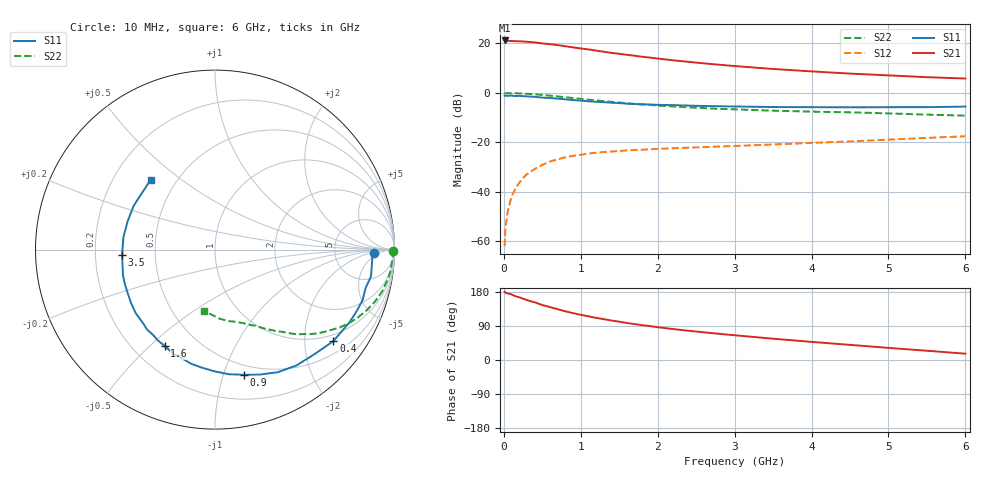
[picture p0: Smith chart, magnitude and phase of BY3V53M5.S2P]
! SIEMENS Small Signal Semiconductors
! BFY420
! Si NPN RF SIEGET Grounded Emitter Transistor in MICRO-X
! VCE = 3.5 V  IC = 3.5 mA
! Common Emitter S-Parameters:  October  1996
# GHz  S  MA  R  50
!  f  S11  S21  S12  S22
! GHz  MAG  ANG  MAG  ANG  MAG  ANG  MAG  ANG
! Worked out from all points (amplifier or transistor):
!   36 points, 10 MHz to 6 GHz, reference 50 ohm
!   highest |S21| = 21.2 dB at 10 MHz (marker M1)
!   |S21| within 3 dB of that: start of sweep to 945.6 MHz
!   unconditionally stable (mu >= 1): 3.471 GHz to end of sweep
!   at 250 MHz: K = 0.10, MSG = 27.6 dB, |S12| = -34.4 dB
!   at 1.4 GHz: K = 0.42, MSG = 19.9 dB, |S12| = -23.7 dB
!   at 6 GHz: K = 1.17, MAG = 9.2 dB, |S12| = -17.5 dB
!   S11 on the Smith chart (normalised r, x): 10 MHz: 16, -3; 400 MHz: 0.81, -2.71; 900 MHz: 0.41, -1.17; 1.6 GHz: 0.33, -0.56; 3.5 GHz: 0.32, -0.03; 6 GHz: 0.36, +0.39
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0.01  0.8833 -1.2  11.48 180.0  0.0008 66.2  0.9937 -0.5
0.02  0.878 -2.2  11.46 177.9  0.0018 66.5  0.9854 -0.8
0.05  0.8777 -4.7  11.24 175.6  0.004 79.9  0.9914 -2.3
0.1  0.8821 -9.7  11.2 173.0  0.008 83.2  0.9868 -4.7
0.15  0.8661 -14.3  11.12 168.3  0.0117 79.7  0.9847 -7.0
0.2  0.8691 -19.1  11.05 165.6  0.0152 77.5  0.9782 -9.3
0.3  0.8512 -28.5  10.8 158.2  0.0228 73.9  0.9613 -13.8
0.4  0.8336 -37.7  10.48 152.3  0.0289 69.2  0.9369 -18.1
0.5  0.8045 -46.3  10 145.0  0.0351 65.4  0.9095 -21.9
0.6  0.7894 -54.8  9.654 139.6  0.0411 61.0  0.8799 -25.6
0.7  0.7674 -62.9  9.249 134.0  0.0454 57.3  0.8496 -29.0
0.9  0.7161 -76.9  8.32 123.6  0.0535 51.2  0.7866 -34.7
1.1  0.6781 -90.3  7.566 115.2  0.0595 46.2  0.7318 -39.7
1.4  0.6334 -106.8  6.424 104.2  0.0653 41.2  0.6616 -45.5
1.6  0.6057 -117.6  5.882 97.6  0.0689 38.3  0.6179 -48.7
2  0.5736 -134.3  4.951 86.5  0.0741 34.4  0.5555 -54.1
2.2  0.5662 -141.2  4.564 81.7  0.0762 33.1  0.5335 -56.5
2.8  0.5376 -159.2  3.712 69.1  0.0826 30.9  0.476 -62.7
3.5  0.5186 -176.7  3.047 56.2  0.0908 29.4  0.438 -69.2
4.5  0.5117 162.1  2.456 39.9  0.1048 27.3  0.405 -79.4
5.5  0.5154 141.6  2.079 24.4  0.1234 24.0  0.3644 -92.5
6  0.5294 132.5  1.953 16.7  0.133 21.6  0.3464 -100.3
